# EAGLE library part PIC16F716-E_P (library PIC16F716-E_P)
8-bit Flash-based Microcontroller Source: Datasheet
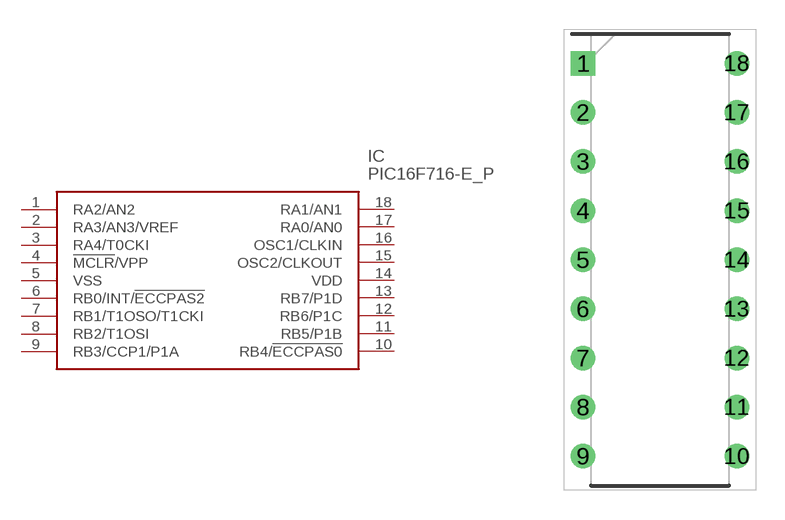
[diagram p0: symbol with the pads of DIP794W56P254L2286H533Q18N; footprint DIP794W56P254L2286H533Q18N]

Designator prefix IC

## PIC16F716-E_P (Description: 8-bit Flash-based Microcontroller; Height: 5.334mm; Manufacturer_Name: Microchip; Manufacturer_Part_Number: PIC16F716-E/P; Mouser_Part_Number: 579-PIC16F716-E/P; Mouser_Price-Stock: https://www.mouser.co.uk/ProductDetail/Microchip-Technology-Atmel/PIC16F716-E-P?qs=JmwSjbzn2OJrC1fbWCIrog%3D%3D)  [DIP794W56P254L2286H533Q18N]
1  RA2/AN2
2  RA3/AN3/VREF
3  RA4/T0CKI
4  !MCLR!/VPP
5  VSS
6  RB0/INT/!ECCPAS2
7  RB1/T1OSO/T1CKI
8  RB2/T1OSI
9  RB3/CCP1/P1A
10  RB4/!ECCPAS0
11  RB5/P1B
12  RB6/P1C
13  RB7/P1D
14  VDD
15  OSC2/CLKOUT
16  OSC1/CLKIN
17  RA0/AN0
18  RA1/AN1

## Footprint DIP794W56P254L2286H533Q18N (pad centres in mm)
12
drill 0.759 pad 1.159 square: 1 -3.969,10.16
drill 0.759 pad 1.159: 2 -3.969,7.62; 3 -3.969,5.08; 4 -3.969,2.54; 5 -3.969,0; 6 -3.969,-2.54; 7 -3.969,-5.08; 8 -3.969,-7.62; 9 -3.969,-10.16; 10 3.969,-10.16; 11 3.969,-7.62; 12 3.969,-5.08; 13 3.969,-2.54; 14 3.969,0; 15 3.969,2.54; 16 3.969,5.08; 17 3.969,7.62; 18 3.969,10.16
